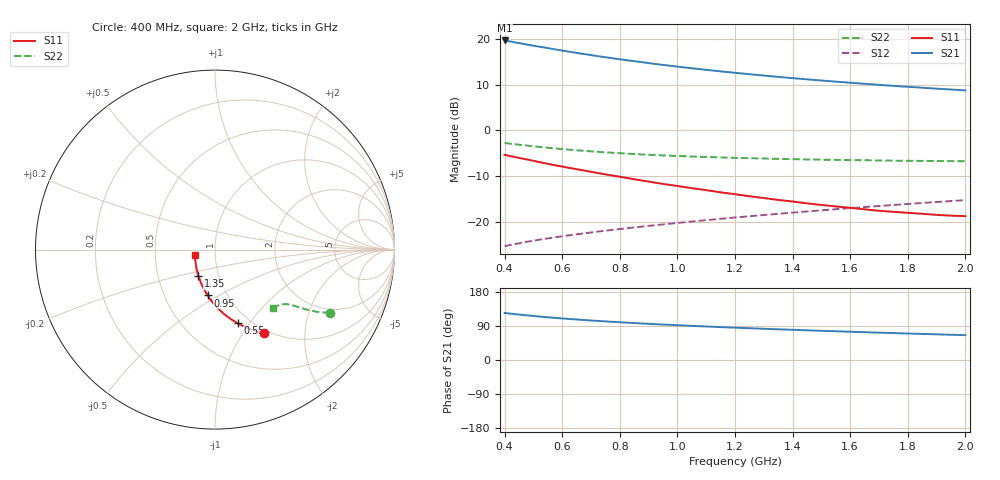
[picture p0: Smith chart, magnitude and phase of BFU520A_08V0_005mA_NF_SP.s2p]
! Filename:  P:\Prog\Test\Noise\ATS_data\Testdata_Net\06 Compressed Noise after Statistics\BFU520A_APG2013_30_A05_08p0V_005mA_NF_CM01_D.sf
! Date/Time: Wed 24/Apr/2013 20:06:19
! BFU520A_APG2013_30_A05_08p0V_1to20mA_NF_CM01_Bias4_R.sf
! Noise Parameter Data File
! BFU520A_APG2013_30_A05_08p0V_1to20mA_NF_CM01
! Date/time: Thu Apr 11 09:33:54 2013
! VAR V_out= 8.000000
! VAR I_out= 5.000000
! VAR V_in= 0.823400
! VAR I_in= 0.053105
! Device data file deembeded for feedlines and parallel
! Original file: \06 Compressed Noise after Statistics\BFU520A_APG2013_30_A05_08p0V_005mA_NF_CM01_R.sf
! Feed-files: PR017V01_150413_Feed1.s2p, PR017V01_150413_Feed2.s2p
! Parallel-file: PR017V01_150413_Par.s2p
# MHz S MA R 50
!  Freq-MHz  S11-mag  S11-arg  S21-mag  S21-arg  S12-mag  S12-arg  S22-mag  S22-arg
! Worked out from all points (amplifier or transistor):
!   37 points, 400 MHz to 2 GHz, reference 50 ohm
!   highest |S21| = 19.8 dB at 400 MHz (marker M1)
!   |S21| within 3 dB of that: start of sweep to 677.7 MHz
!   unconditionally stable (mu >= 1): 1.658 GHz to end of sweep
!   at 500 MHz: K = 0.62, MSG = 21.4 dB, |S12| = -24.2 dB
!   at 1.1 GHz: K = 0.92, MSG = 16.5 dB, |S12| = -19.7 dB
!   at 2 GHz: K = 1.01, MAG = 11.4 dB, |S12| = -15.3 dB
!   lowest NFmin = 0.65 dB at 420 MHz
!   S11 on the Smith chart (normalised r, x): 400 MHz: 0.96, -1.25; 550 MHz: 0.87, -0.88; 950 MHz: 0.81, -0.45; 1.35 GHz: 0.80, -0.24; 2 GHz: 0.80, -0.04
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400  0.5383 -59.4  9.719 124.1  0.05361 65.0  0.7282 -28.8
420  0.5223 -61.4  9.461 122.3  0.05531 64.6  0.7153 -29.4
440  0.5066 -63.4  9.216 120.7  0.05696 64.3  0.7033 -29.9
480  0.478 -67.0  8.732 117.7  0.06008 63.8  0.68 -30.8
500  0.4635 -68.8  8.513 116.2  0.06164 63.6  0.6699 -31.2
550  0.4295 -72.9  8.013 112.7  0.06522 63.2  0.6443 -32.1
600  0.4007 -76.7  7.526 109.6  0.06885 63.0  0.6237 -32.8
650  0.3754 -80.2  7.096 106.9  0.07236 63.0  0.6054 -33.4
700  0.3512 -83.6  6.712 104.2  0.0758 63.0  0.5891 -33.8
750  0.3293 -86.8  6.355 101.8  0.07926 63.1  0.5747 -34.2
800  0.31 -90.1  6.039 99.6  0.0827 63.2  0.5621 -34.6
850  0.291 -93.1  5.75 97.5  0.08614 63.4  0.5508 -35.0
900  0.2746 -96.2  5.485 95.5  0.08959 63.5  0.5409 -35.4
950  0.2587 -99.0  5.241 93.6  0.09299 63.7  0.5319 -35.7
1050  0.2323 -104.7  4.812 90.1  0.09993 64.2  0.5168 -36.4
1100  0.221 -107.7  4.625 88.4  0.1035 64.3  0.5108 -36.7
1200  0.1995 -113.5  4.29 85.3  0.1106 64.7  0.4998 -37.4
1350  0.1726 -122.3  3.87 81.0  0.1215 65.0  0.4874 -38.6
1500  0.152 -131.8  3.531 77.1  0.1327 65.3  0.4772 -40.0
1650  0.1361 -141.6  3.25 73.4  0.1442 65.3  0.4705 -41.5
1750  0.1278 -148.6  3.085 71.0  0.1518 65.4  0.4657 -42.6
2000  0.1146 -166.2  2.752 65.6  0.1717 65.1  0.4587 -45.6
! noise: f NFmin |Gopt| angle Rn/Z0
400  0.6987  0.2137  9.63  0.137
460  0.6671  0.1841  19.12  0.1249
600  0.7544  0.1884  22.26  0.1447
800  0.7211  0.1749  38.02  0.1175
1000  0.765  0.1632  52.05  0.1111
1200  0.7967  0.1565  62.85  0.1107
1400  0.8295  0.1329  77.69  0.1041
1600  0.8277  0.1318  99.57  0.0941
1800  0.8207  0.1534  140.3  0.0714
2000  0.8217  0.1049  145.9  0.0875
